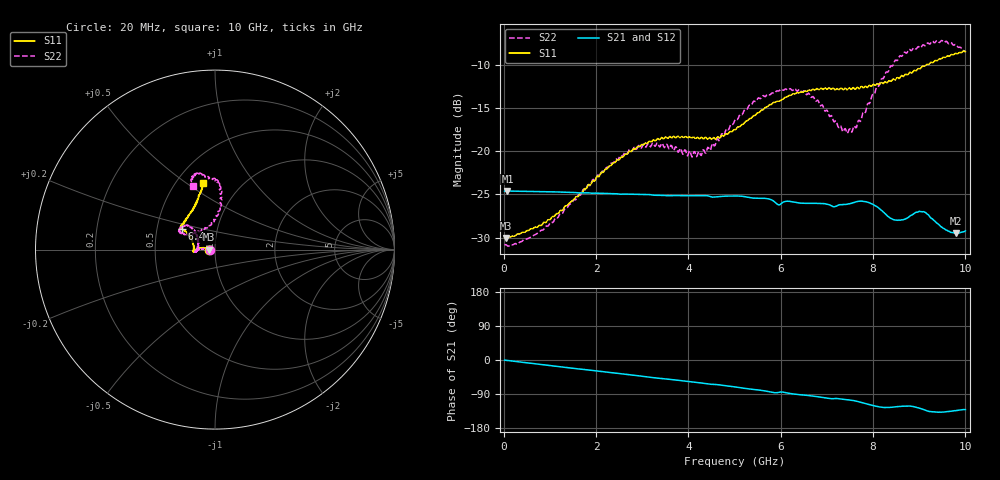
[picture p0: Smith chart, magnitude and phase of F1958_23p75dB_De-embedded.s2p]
! Integrated Device Technology
! Corporate Headquarters
! 6024 Silver Creek Valley Road
! San Jose, CA 95138  USA
! Phone:  1-408-284-8200
! Toll Free:  1-800-223-1366
! Webpage:  http://www.idt.com/
! Timing and RF Division
! 515 Groton Road, Suite 102
! Westford, MA 01886-6024
! Device:  F1958
! Description: 7-bit 0.25 dB Digital Step Attenuator
! Frequency:  0.001 -  6.000 GHz
! Package:  4x4 mm Thin QFN Plastic Package: 24 pin
! Ports:  2 RF, 12 DC
!  Pin  1  = D0
!  Pin  2  = VDD
!  Pin  3  = VMODE
!  Pin  4  = GND
!  Pin  5  = RF1  =  Port 1
!  Pin  6  = GND
!  Pin  7  = GND
!  Pin  8  = GND
!  Pin  9  = GND
!  Pin 10  = GND
!  Pin 11  = GND
!  Pin 12  = GND
!  Pin 13  = GND
!  Pin 14  = RF2  =  Port 2
!  Pin 15  = GND
!  Pin 16  = LE
!  Pin 17  = CLK
!  Pin 18  = DATA
!  Pin 19  = D6
!  Pin 20  = D5
!  Pin 21  = D4
!  Pin 22  = D3
!  Pin 23  = D2
!  Pin 24  = D1
! State:  95
! Atten State:  23.75 dB
! Voltage:  +3.30 Volts
! Current:  0.258 mA
! Data:  The device was measured on a F1958 evaluation board which has
!  individual transmission lines to the RF pins.  Data was collected
!  using a calibrated network analyzer.  The evaluation board was
!  de-embedded using Automatic Fixture Removal (AFR).
!  The reference plane is the edge of the package pin.
! Misc:
!  Action Tracker AT0419
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# GHz S dB R 50
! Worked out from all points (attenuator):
!   500 points, 20 MHz to 10 GHz, reference 50 ohm
!   highest |S21| = -24.61 dB at 80 MHz (marker M1); lowest = -29.5 dB at 9.8 GHz (marker M2)
!   lowest |S11| = -30.1 dB at 40 MHz (marker M3), VSWR 1.06, Z = 47 - j0.0422 ohm
!   |S11| at or under -10 dB: start of sweep to 9.15 GHz
!   |S22| runs from -31.0 to -7.2 dB; largest |S21 - S12| = 0.00037
!   S11 on the Smith chart (normalised r, x): 20 MHz: 0.94, -0.00; 6.4 GHz: 0.67, +0.16; 10 GHz: 0.67, +0.58
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0.02  -30.03 -178.9  -24.62 -0.4  -24.61 -0.3  -30.85 -178.8
0.04  -30.05 -179.2  -24.61 -0.6  -24.61 -0.6  -30.82 -178.2
0.08  -29.97 179.4  -24.61 -1.2  -24.61 -1.2  -30.96 -178.3
0.84  -28.45 170.7  -24.69 -12.3  -24.68 -12.2  -29.14 176.5
1.7  -24.80 170.7  -24.83 -24.4  -24.82 -24.4  -24.68 174.9
2.62  -20.40 176.8  -24.97 -37.4  -24.95 -37.4  -20.14 -179.0
3.36  -18.64 -175.8  -25.11 -48.0  -25.12 -48.2  -19.36 -171.8
4.24  -18.57 -179.2  -25.15 -60.0  -25.16 -60.1  -20.07 166.3
4.64  -18.33 171.6  -25.27 -65.3  -25.28 -65.3  -18.58 148.4
5.02  -17.50 160.7  -25.18 -71.2  -25.19 -71.2  -16.28 138.0
5.58  -15.24 150.5  -25.46 -80.1  -25.47 -80.1  -13.82 138.5
6.4  -13.24 147.9  -26.00 -91.5  -26.02 -91.4  -12.83 152.1
6.68  -12.88 146.8  -26.03 -95.0  -26.05 -94.8  -13.73 153.0
7.3  -12.69 141.1  -26.20 -102.9  -26.20 -102.8  -17.06 132.5
7.5  -12.72 138.5  -26.08 -105.7  -26.08 -105.7  -17.42 114.4
7.9  -12.49 129.3  -25.93 -117.0  -25.92 -117.1  -14.44 88.2
8.34  -11.86 119.3  -27.60 -125.4  -27.61 -125.5  -10.67 82.7
8.66  -11.36 113.6  -27.94 -121.9  -27.94 -121.8  -8.68 85.9
9.08  -10.13 107.6  -27.01 -130.3  -27.02 -130.3  -7.68 96.3
9.4  -9.48 102.8  -28.39 -137.9  -28.41 -137.9  -7.22 104.2
9.8  -8.68 101.0  -29.50 -133.4  -29.53 -133.3  -7.67 108.8
10  -8.47 100.1  -29.22 -131.0  -29.25 -130.8  -8.46 109.2
